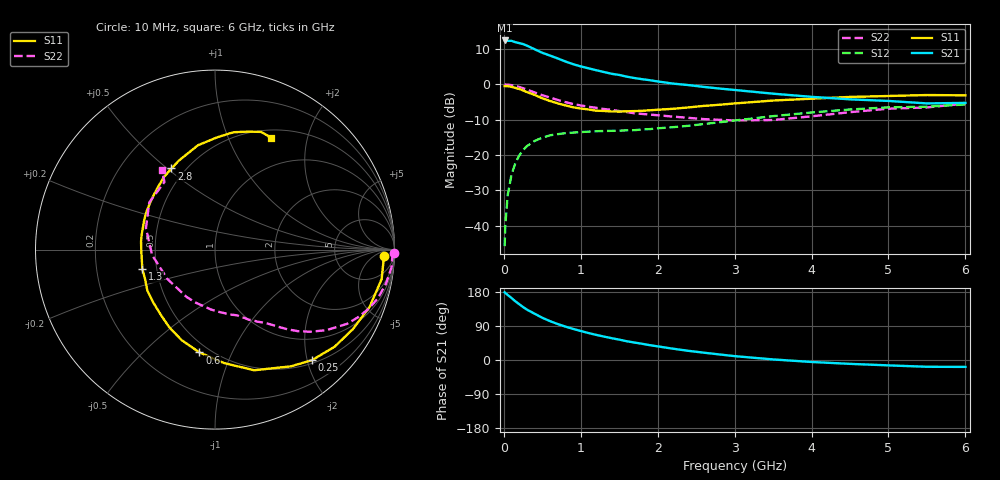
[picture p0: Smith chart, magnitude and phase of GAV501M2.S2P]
! Infineon Technologies  Discrete & RF Semiconductors
! BF775
! Si NPN RF Bipolar Junction Transistor in SOT23
! VCE = 0.5 V  IC = 1.2 mA
! Common Emitter S-Parameters:  May  1996
# GHz  S  MA  R  50
!  f  S11  S21  S12  S22
! GHz  MAG  ANG  MAG  ANG  MAG  ANG  MAG  ANG
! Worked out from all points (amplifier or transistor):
!   36 points, 10 MHz to 6 GHz, reference 50 ohm
!   highest |S21| = 12.4 dB at 10 MHz (marker M1)
!   |S21| within 3 dB of that: start of sweep to 450.9 MHz
!   unconditionally stable (mu >= 1): 1.211 GHz to end of sweep
!   at 250 MHz: K = 0.25, MSG = 15.0 dB, |S12| = -18.7 dB
!   at 1.4 GHz: K = 1.11, MAG = 6.0 dB, |S12| = -13.2 dB
!   at 6 GHz: K = 1.12, MAG = -1.9 dB, |S12| = -5.7 dB
!   S11 on the Smith chart (normalised r, x): 10 MHz: 24, -15; 250 MHz: 0.56, -2.09; 600 MHz: 0.44, -0.76; 1.3 GHz: 0.42, -0.11; 2.8 GHz: 0.42, +0.52; 6 GHz: 0.60, +1.45
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0.01  0.9414 -2.1  4.175 178.7  0.0051 87.8  0.9967 -1.1
0.02  0.9409 -4.1  4.135 176.6  0.0104 85.6  0.9889 -2.3
0.05  0.943 -10.0  4.124 171.8  0.0269 83.3  0.9885 -5.7
0.1  0.919 -20.2  4.123 163.6  0.0526 77.9  0.972 -11.1
0.15  0.8873 -29.9  3.948 154.8  0.0765 70.9  0.9472 -16.7
0.25  0.8194 -48.7  3.712 139.7  0.1168 60.4  0.8797 -25.5
0.3  0.7761 -56.9  3.524 133.0  0.1332 56.0  0.8434 -29.4
0.4  0.7069 -72.0  3.134 122.1  0.1576 48.1  0.7656 -35.9
0.5  0.6339 -85.5  2.793 111.4  0.1756 42.0  0.7006 -40.8
0.6  0.5793 -98.6  2.551 102.6  0.1892 37.3  0.6485 -44.5
0.7  0.5377 -110.2  2.323 94.9  0.1968 33.6  0.6005 -47.7
0.8  0.5015 -120.7  2.104 88.1  0.203 30.7  0.5595 -50.4
0.9  0.4726 -129.6  1.926 82.1  0.2069 28.7  0.5252 -52.9
1.1  0.4401 -149.0  1.685 71.2  0.2137 25.5  0.4808 -57.4
1.3  0.4191 -165.1  1.493 61.9  0.2182 23.6  0.4467 -61.7
1.7  0.4174 167.4  1.225 46.0  0.2239 24.5  0.3874 -71.2
2.2  0.4499 142.1  1.023 29.8  0.2469 26.2  0.3485 -86.0
2.8  0.513 118.2  0.871 14.7  0.2895 27.0  0.3141 -110.8
3.5  0.5889 99.3  0.736 1.5  0.354 23.3  0.3119 -148.4
4.5  0.6622 81.0  0.612 -10.2  0.4399 12.9  0.403 162.7
5.5  0.7043 68.6  0.536 -17.9  0.4817 -0.5  0.4701 126.8
6  0.6976 63.3  0.545 -18.2  0.5185 -4.1  0.5338 123.6
